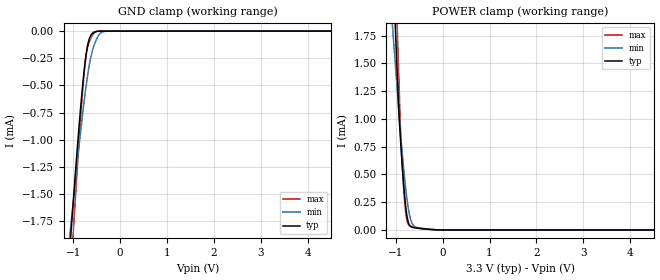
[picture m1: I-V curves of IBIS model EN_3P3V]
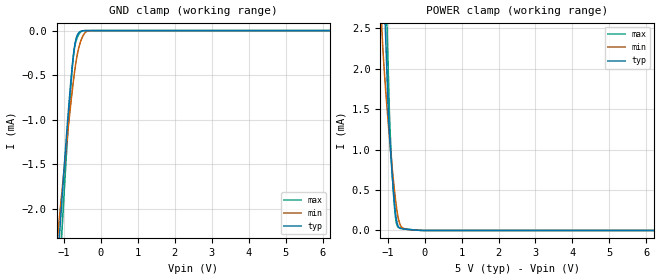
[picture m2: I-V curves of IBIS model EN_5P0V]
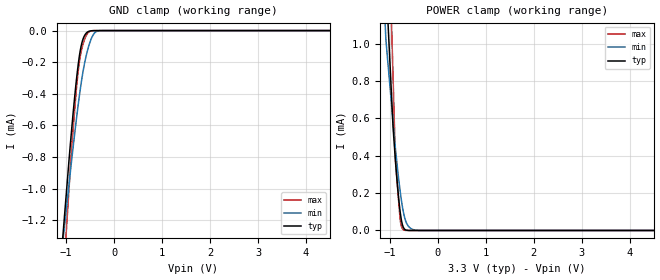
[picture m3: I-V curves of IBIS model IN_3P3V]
| Texas Instruments Incorporated
| Low-Power Quad-channel Digital Isolator
| Marketing part#   Voltage Range   Package-type   #pins/pkg drawing
| ISO7341FCDW   3.0V - 5.5V   SOIC   16-pin DW
| ISO7341FCDWR   3.0V - 5.5V   SOIC   16-pin DW
[IBIS Ver]   4.1
[File name]   iso7341fc.ibs
[File Rev]   1.0
[Date]   09/30/2014
[Source]   Model built from spectre simulations at:
   Texas Instruments Incorporated.
   Analog-eLab, HPA
   12500 TI Blvd
   Dallas, TX -75243
   For Support e-mail: elab_ibis@list.ti.com
[Notes]   Revision History
   Rev 1.0: 09/30/2014
   - GND Clamp non monotonic for EN and IN input buffers
   - ccomp values are based on PVT settings:
   MIN: Low Voltage, High Temperature, Weak Process
   TYP: Nominal Voltage, Nominal Temperature, Nominal Process
   MAX: High Voltage, Low Temperature, Fast Process
   - C_comp although listed in numerical order of value are obtained from varying PVT conditions.
   For PVT conditions for each specific value, refer to the buffer description under respective [Model].
   IBIS model user is responsible for using appropriate C_comp to simulate for Signal Integrity.
[Disclaimer]  This model is designed as an aid for customers of Texas Instruments
 TI and its licensors and suppliers make no warranties, either expressed
 or implied, with respect to this  model, including the warranties of
 merchantability or fitness for a particular purpose.
 The model is provided solely on an "as is" basis. The entire risk as to
 its quality and performance is with the customer.
[Copyright] (C)Copyright 2014 Texas Instruments Incorporated.
   All rights reserved.
[Component]   ISO7341FCDW
[Manufacturer]  Texas Instruments Incorporated
[Package]   |16-pin SOIC DW package
|   typ   min   max
R_pkg   0.1228   0.0822   0.1793
L_pkg   2.2157n   1.9245n   2.8571n
C_pkg   0.4645p   0.2145p   0.7510p
[Pin]   signal_name   model_name   R_pin   L_pin   C_pin
1   VCC1   POWER   0.09703  2.25823n  0.63889p
2   GND1   GND   0.10567  2.15194n  0.30706p
3   INA   IN   0.12889  1.99554n  0.21450p
4   INB   IN   0.12623  1.94755n  0.61276p
5   INC   IN   0.12494  1.92646n  0.36666p
6   OUTD   OUT   0.14038  2.18765n  0.43235p
7   EN1   EN   0.17807  2.83638n  0.45904p
8   GND1   GND   0.08216  2.43955n  0.44498p
9   GND2   GND   0.10126  2.44074n  0.40934p
10   EN2   EN   0.17928  2.85707n  0.52717p
11   IND   IN   0.12883  1.99615n  0.50841p
12   OUTC   OUT   0.12617  1.94399n  0.32633p
13   OUTB   OUT   0.12498  1.92454n  0.37783p
14   OUTA   OUT   0.14050  2.18615n  0.38097p
15   GND2   GND   0.08275  2.09014n  0.75096p
16   VCC2   POWER   0.09747  2.26909n  0.67439p
[Model Selector] IN
IN_3P3V   3.3V Input
IN_5P0V   5.0V Input
[Model Selector] EN
EN_3P3V   3.3V Input
EN_5P0V   5.0V Input
[Model Selector] OUT
OUT_3P3V   3.3V Output
OUT_5P0V   5.0V Output
| Models and submodels in the file (6): EN_3P3V (Input), EN_5P0V (Input), IN_3P3V (Input), IN_5P0V (Input), OUT_3P3V (3-state), OUT_5P0V (3-state)
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|   Model EN_3P3V
[Model]   EN_3P3V
Model_type   Input
Vinl = .8
Vinh = 2
|   typ   min   max
|   (nom PVT)   (slow PVT)   (fast PVT)
C_comp   0.161p   0.098p   0.252p
| Where   nom PVT is  Nominal Process, 3.3V, 27C
|   Fast PVT is Strong Process, 3.6V, -40C
|   Slow PVT is Weak Process, 3.0V, 150C
[Voltage Range]   3.3   3   3.6
[Temperature Range]   27   150   -40
[Power Clamp Reference]   3.3   3   3.6
[GND Clamp Reference]   0   0   0
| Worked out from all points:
|   GND clamp passes 1 mA (typ) near -0.90 V on its own axis
|   POWER clamp passes 1 mA (typ) near -0.92 V on its own axis
[GND Clamp]
|   Voltage   I(typ)   I(min)   I(max)
-3.3V     -16.02mA   -12.12mA   -20.07mA
-1.082V   -2.058mA   -1.927mA   -2.435mA
-933.9mV  -1.195mA   -1.301mA   -1.409mA
-815.1mV  -576.9uA   -823.1uA   -642.6uA
-775.5mV  -399.7uA   -677.1uA   -429.5uA
-735.9mV  -249.5uA   -540.6uA   -261.7uA
-696.3mV  -138.4uA   -417.2uA   -157.1uA
-656.7mV  -70.87uA   -311.6uA   -97.71uA
-547.8mV  -8.269uA   -122.2uA   -15.56uA
-438.9mV  -609.9nA   -28.59uA   -715.7nA
-300.3mV  -135.4nA   -1.693uA   -73.15nA
6.6V      0A         0A         0A
[POWER Clamp]
|   Voltage   I(typ)   I(min)   I(max)
-3.3V     37.87mA    27.97mA    46.61mA
-1.082V   2.59mA     1.912mA    3.362mA
-933.9mV  1.066mA    1.077mA    1.378mA
-894.3mV  792.6uA    854.2uA    848.9uA
-844.8mV  490.1uA    618.8uA    468.6uA
-795.3mV  245.9uA    408.6uA    190uA
-765.6mV  141.6uA    299.7uA    94.29uA
-735.9mV  76.12uA    208uA      52.02uA
-656.7mV  25.39uA    64.33uA    30.38uA
-518.1mV  15.3uA     15.27uA    20.19uA
-3.3mV    22.97nA    56.83nA    14.08nA
6.6V      0A         0A         0A
|   Model EN_5P0V
[Model]   EN_5P0V
Model_type   Input
Vinl = .8
Vinh = 2
|   typ   min   max
|   (nom PVT)   (slow PVT)   (fast PVT)
C_comp   0.173p   0.101p   0.247p
| Where   nom PVT is  Nominal Process, 5.0V, 27C
|   Fast PVT is Strong Process, 5.5V, -40C
|   Slow PVT is Weak Process, 4.5V, 150C
[Voltage Range]   5   4.5   5.5
[Temperature Range]   27   150   -40
[Power Clamp Reference]   5   4.5   5.5
[GND Clamp Reference]   0   0   0
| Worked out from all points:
|   GND clamp passes 1 mA (typ) near -0.90 V on its own axis
|   POWER clamp passes 1 mA (typ) near -0.92 V on its own axis
[GND Clamp]
|   Voltage   I(typ)   I(min)   I(max)
-5V       -26.85mA   -20.05mA   -33.83mA
-1.235V   -2.983mA   -2.6mA     -3.546mA
-1.13V    -2.354mA   -2.134mA   -2.795mA
-1.115V   -2.264mA   -2.068mA   -2.688mA
-1.055V   -1.904mA   -1.808mA   -2.259mA
-860mV    -799.2uA   -997uA     -914.7uA
-755mV    -317.8uA   -605uA     -335.4uA
-665mV    -81.82uA   -332uA     -109.5uA
-530mV    -5.449uA   -101.8uA   -10.68uA
-425mV    -437.8nA   -22.05uA   -447nA
-275mV    -117.8nA   -1.166uA   -60.6nA
10V       0A         0A         0A
[POWER Clamp]
|   Voltage   I(typ)   I(min)   I(max)
-5V       66.01mA    49.38mA    80.54mA
-1.235V   4.734mA    3.205mA    6.08mA
-1.13V    3.373mA    2.244mA    4.359mA
-1.085V   2.789mA    1.93mA     3.621mA
-1.055V   2.4mA      1.739mA    3.129mA
-1.025V   2.011mA    1.559mA    2.638mA
-980mV    1.427mA    1.304mA    1.9mA
-935mV    1.075mA    1.063mA    1.241mA
-845mV    491.9uA    621.1uA    470.4uA
-770mV    155.2uA    316.2uA    105.1uA
-650mV    24.69uA    59.36uA    30.24uA
10V       0A         0A         0A
|   IN_3P3V Model
[Model]   IN_3P3V
Model_type   Input
Vinl = 0.8
Vinh = 2
|   typ   min   max
|   (nom PVT)   (slow PVT)   (fast PVT)
C_comp   0.351pF   0.323pF   0.382pF
| Where   nom PVT is  Nominal Process, 3.3V, 27C
|   Fast PVT is Strong Process, 3.6V, -40C
|   Slow PVT is Weak Process, 3.0V, 150C
[Voltage Range]   3.3   3   3.6
[Temperature Range]   27   150   -40
[Power Clamp Reference]   3.3   3   3.6
[GND Clamp Reference]   0   0   0
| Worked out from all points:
|   GND clamp passes 1 mA (typ) near -0.99 V on its own axis
|   POWER clamp passes 1 mA (typ) near -1.02 V on its own axis
[GND Clamp]
|   Voltage   I(typ)   I(min)   I(max)
-3.3V     -10.39mA   -8.115mA   -12.82mA
-1.082V   -1.354mA   -1.374mA   -1.677mA
-933.9mV  -797.4uA   -956.1uA   -972uA
-884.4mV  -624.8uA   -817.9uA   -737uA
-785.4mV  -312.4uA   -559.5uA   -368.1uA
-735.9mV  -187.2uA   -440.5uA   -225.5uA
-696.3mV  -112uA     -353.2uA   -148.2uA
-646.8mV  -53.31uA   -257.7uA   -85.46uA
-528mV    -5.031uA   -97.34uA   -9.656uA
-419.1mV  -267.9nA   -19.35uA   -326.7nA
-260.7mV  0A         -360nA     0A
6.6V      0A         0A         0A
[POWER Clamp]
|   Voltage   I(typ)   I(min)   I(max)
-3.3V     19.39mA    14.36mA    23.85mA
-1.132V   1.605mA    1.287mA    2.629mA
-1.082V   1.342mA    1.019mA    2.178mA
-933.9mV  554.7uA    582.1uA    822.8uA
-884.4mV  378uA      439.9uA    371.2uA
-834.9mV  221.9uA    318uA      214.3uA
-785.4mV  99.44uA    209.9uA    57.41uA
-745.8mV  38.13uA    138uA      13.04uA
-706.2mV  10.91uA    83.53uA    2.199uA
-607.2mV  297.1nA    20.73uA    21.59nA
-419.1mV  0A         493.2nA    0A
6.6V      0A         0A         0A
